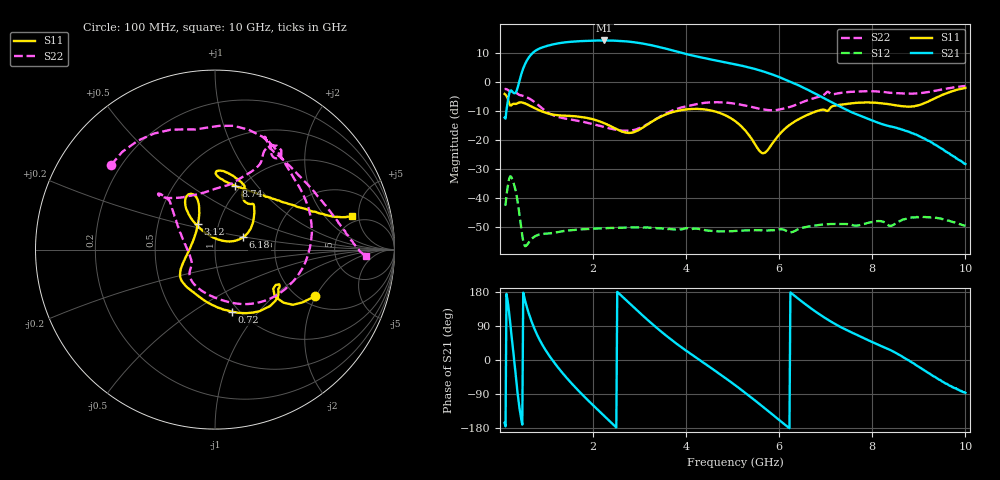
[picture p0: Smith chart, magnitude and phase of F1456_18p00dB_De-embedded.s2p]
! Integrated Device Technology
! Corporate Headquarters
! 6024 Silver Creek Valley Road
! San Jose, CA 95138  USA
! Phone:  1-408-284-8200
! Toll Free:  1-800-223-1366
! Webpage:  http://www.idt.com/
! Timing and RF Division
! 515 Groton Road, Suite 102
! Westford, MA 01886-6024
! Device:  F1456
! Description: 6-bit 0.5 dB Transmit Variable Gain Amplifier
! Frequency:  2100.0 -  2950.00 MHz
! Package:  6x6 mm Thin QFN Plastic Package: 28 pin
! State:  36
! Atten State:  18.0 dB
! Voltage:  +5.00 Volts
! Current:  216.996 mA
! Data:  The device was measured on a the F1455 evaluation board which has
!  individual transmission lines to the RF pins.  Data was collected
!  using a calibrated network analyzer.  The evaluation board was
!  de-embedded using a TRL calibration technique.
!  The reference plane is the edge of the package pin.
!  Pin  1 = CSb
!  Pin  2 = DATA
!  Pin  3 = CLK
!  Pin  4 = RSET
!  Pin  5 = GND
!  Pin  6 = RFIN  = Port 1
!  Pin  7 = GND
!  Pin  8 = NC
!  Pin  9 = NC
!  Pin 10 = NC
!  Pin 11 = NC
!  Pin 12 = NC
!  Pin 13 = NC
!  Pin 14 = /STBY
!  Pin 15 = GND
!  Pin 16 = RFOUT  = Port 2
!  Pin 17 = GND
!  Pin 18 = NC
!  Pin 19 = NC
!  Pin 20 = NC
!  Pin 21 = GND
!  Pin 22 = NC
!  Pin 23 = GND
!  Pin 24 = NC
!  Pin 25 = NC
!  Pin 26 = NC
!  Pin 27 = GND
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# GHz S dB R 50
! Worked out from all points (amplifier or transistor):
!   496 points, 100 MHz to 10 GHz, reference 50 ohm
!   highest |S21| = 14.2 dB at 2.24 GHz (marker M1)
!   |S21| within 3 dB of that: 819.8 MHz to 3.61 GHz (2.79 GHz wide, 126 % of centre)
!   unconditionally stable (mu >= 1): start of sweep to end of sweep
!   at 1.74 GHz: K = 31.11, MAG = 14.4 dB, |S12| = -50.8 dB
!   at 5.06 GHz: K = 72.93, MAG = 7.0 dB, |S12| = -51.3 dB
!   at 10 GHz: K = 429.69, MAG = -18.7 dB, |S12| = -49.6 dB
!   S11 on the Smith chart (normalised r, x): 100 MHz: 2.36, -1.99; 720 MHz: 0.93, -0.74; 3.12 GHz: 0.80, +0.24; 6.18 GHz: 1.35, +0.19; 8.74 GHz: 0.94, +0.78; 10 GHz: 4.20, +4.09
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0.1  -4.19 -25.0  -12.34 -165.8  -42.33 48.6  -2.54 140.8
0.3  -7.61 -30.9  -3.93 6.4  -35.24 -133.0  -3.17 74.4
0.42  -7.13 -37.9  0.41 -127.2  -45.83 140.7  -4.55 41.9
0.56  -7.62 -56.5  6.74 147.5  -56.45 154.6  -5.21 10.3
0.72  -8.88 -74.5  10.12 88.7  -53.52 139.4  -6.74 -25.2
0.96  -10.56 -98.1  12.06 30.0  -52.27 95.4  -9.84 -68.7
1.18  -11.43 -114.9  12.97 -9.1  -51.88 71.2  -11.74 -95.2
1.48  -11.74 -131.1  13.67 -53.7  -51.12 47.0  -12.89 -119.7
1.76  -12.14 -141.7  13.98 -90.2  -50.72 29.4  -13.71 -132.7
2.24  -14.27 -157.1  14.19 -147.6  -50.35 5.0  -15.56 -143.6
2.64  -17.24 174.4  13.97 165.9  -50.21 -14.1  -16.84 -157.6
3.12  -15.25 123.0  12.98 111.5  -50.10 -37.6  -15.05 166.2
3.4  -12.49 111.7  12.02 81.6  -50.39 -50.6  -12.39 148.4
3.72  -10.42 109.4  10.73 49.9  -50.82 -64.2  -9.80 137.0
4.08  -9.41 113.3  9.21 17.8  -50.66 -80.3  -8.19 133.1
5.06  -13.61 127.4  5.97 -67.1  -51.30 -125.5  -7.57 135.2
5.66  -24.59 70.2  3.53 -124.5  -51.18 -160.7  -9.54 116.9
6.18  -15.38 23.7  0.36 -176.1  -51.49 165.6  -8.87 80.7
6.7  -10.77 41.2  -3.48 134.7  -49.60 143.0  -5.90 63.4
8.36  -7.74 88.1  -15.27 28.0  -49.51 69.6  -3.78 62.5
8.74  -8.56 72.2  -16.98 1.8  -47.05 64.9  -4.09 49.2
10  -2.11 13.8  -28.28 -86.6  -49.58 -22.8  -1.46 -2.6
